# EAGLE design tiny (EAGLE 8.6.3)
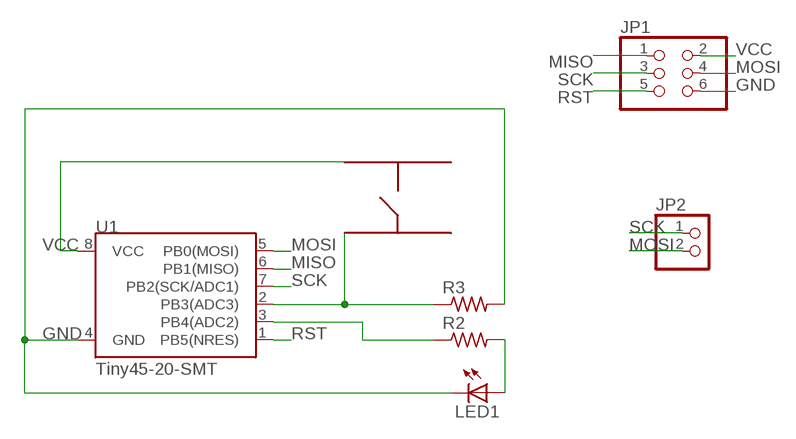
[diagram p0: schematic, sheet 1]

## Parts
JP1  PINHD-2X3  [2X03]
JP2  PINHD-1X2  [1X02]
LED1  LEDCHIPLED_1206  [CHIPLED_1206]
R2  R-US_R1206  [R1206]
R3  R-US_R1206  [R1206]
S1  TACTSWITCH  [TACT]
U1  Tiny45-20-SMT  ATTINY45TINY45-20-SMT  [SO08-EIAJ]

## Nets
GND: JP1.6 LED1.C R3.2 U1.4(GND)
MISO: JP1.1 U1.6(PB1(MISO))
MOSI: JP1.4 JP2.2 U1.5(PB0(MOSI))
N$1: R2.1 U1.3(PB4(ADC2))
N$3: LED1.A R2.2
N$8: R3.1 S1.3 U1.2(PB3(ADC3))
RST: JP1.5 U1.1(PB5(NRES))
SCK: JP1.3 JP2.1 U1.7(PB2(SCK/ADC1))
VCC: JP1.2 S1.1 U1.8(VCC)
Unconnected: S1.2 S1.4

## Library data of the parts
JP1 = pinhead:PINHD-2X3: PIN HEADER
JP2 = pinhead:PINHD-1X2: PIN HEADER
LED1 = led:LED: LED
R2 R3 = resistor:R-US_: RESISTOR, American symbol
S1 = oliver:TACTSWITCH
U1 = SparkFun-DigitalIC:ATTINY45: Atmel 8-pin 2/4/8kB flash uC; PROD_ID: IC-08922

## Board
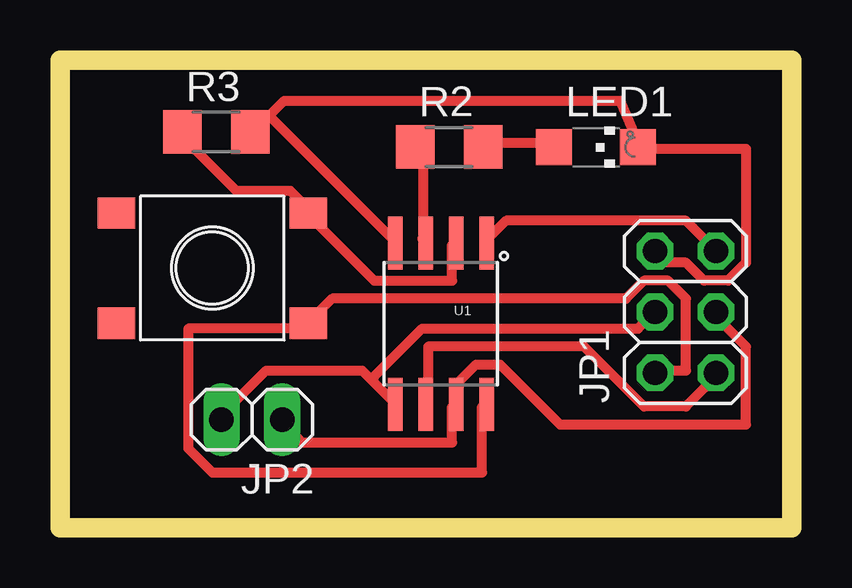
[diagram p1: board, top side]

Size 30.5 x 19.5 mm. Coordinates in mm from the lower left corner, seen from the top.
Outline: 0,0 30.5,0 30.5,19.5 0,19.5 0,0
Copper layers (1*16): Top 0.035mm / dielectric 1.5mm / Bottom 0.035mm
Design rules "default *": minimum track width 16mil, minimum drill 24mil, track to track 10mil, track to pad 10mil, pad to pad 10mil, via to via 10mil, smd to smd 8mil, copper to edge 40mil, drill to drill 8mil, minimum pad ring 10mil, minimum via ring 8mil, stop-mask expansion 4mil, vias tented up to drill 0mil, thermal gap 10mil

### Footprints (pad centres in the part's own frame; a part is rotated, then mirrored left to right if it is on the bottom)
2X03 = drill 1.016 octagon: 1 -2.54,-1.27; 2 -2.54,1.27; 3 0,-1.27; 4 0,1.27; 5 2.54,-1.27; 6 2.54,1.27
1X02 = drill 1.016 long: 1 -1.27,0; 2 1.27,0
CHIPLED_1206 = smd 1.5 x 1.5: A 0,-1.75; C 0,1.75
R1206 = smd 1.6 x 1.803: 1 -1.422,0; 2 1.422,0
TACT = smd 1.55 x 1.3: 1 -4,2.3; 2 4,2.3; 3 -4,-2.3; 4 4,-2.3
SO08-EIAJ = smd 0.61 x 2.21: 1 -1.905,-3.378; 2 -0.635,-3.378; 3 0.635,-3.378; 4 1.905,-3.378; 5 1.905,3.353; 6 0.635,3.353; 7 -0.635,3.353; 8 -1.905,3.353

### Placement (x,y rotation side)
JP1  26.08,8.99 90 top
JP2  8,4.5 180 top
LED1  22.35,15.86 270 top
R2  16.23,15.87 0 top
R3  6.52,16.5 0 top
S1  6.35,10.82 180 top
U1  15.88,8.49 180 top

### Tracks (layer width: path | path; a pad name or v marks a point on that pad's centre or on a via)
GND
  Top 0.406: 8.72,17.18 8.1,16.55 R3.2 | 8.72,17.18 9.35,17.8 23.35,17.8 24.1,16.05 LED1.C 24.1,15.8 28.6,15.8 28.6,11.05 27.85,10.3 26.85,10.3 26.1,11.05 25.1,11.05 24.85,11.3 JP1.6 | U1.4 13.85,12.05 8.85,17.05 8.72,17.18
MISO
  Top 0.406: U1.6 15.35,5.3 15.35,7.55 21.85,7.55 24.35,5.05 26.1,5.05 27.35,6.3 JP1.1
MOSI
  Top 0.406: 12.97,6.17 12.6,6.55 8.6,6.55 6.6,4.55 JP2.2 | 12.97,6.17 13.85,5.3 U1.5 | JP1.4 24.6,8.8 24.1,8.3 15.1,8.3 13.1,6.3 12.97,6.17
N$1
  Top 0.406: R2.1 15.15,15.8 15.15,12.05 15.1,12.05 U1.3
N$3
  Top 0.406: LED1.A 20.6,16.05 17.85,16.05 R2.2
N$8
  Top 0.406: R3.1 5.1,16.3 7.35,14.05 9.6,14.05 10.35,13.3 S1.3 10.35,13.05 13.1,10.3 16.35,10.3 16.35,11.8 U1.2
RST
  Top 0.406: U1.1 17.85,12.05 18.6,12.8 26.1,12.8 27.35,11.55 JP1.5
SCK
  Top 0.406: JP2.1 9.35,4.3 10.1,3.55 16.35,3.55 16.35,5.05 U1.7 16.6,5.3 16.6,6.05 17.35,6.8 18.35,6.8 20.85,4.3 28.6,4.3 28.6,7.55 27.35,8.8 JP1.3
VCC
  Top 0.406: JP1.2 24.85,6.55 26.1,6.55 26.1,9.55 25.35,10.3 24.35,10.3 23.6,9.55 11.35,9.55 10.35,8.55 S1.1 10.35,8.3 5.35,8.3 5.35,3.3 6.35,2.3 17.6,2.3 17.6,5.05 U1.8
